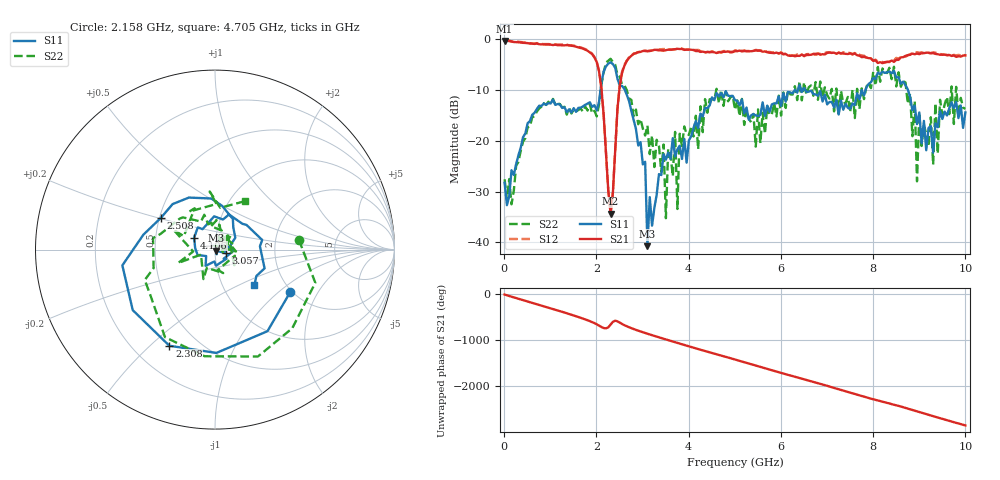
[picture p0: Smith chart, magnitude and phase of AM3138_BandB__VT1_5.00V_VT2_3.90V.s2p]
! Date/Time: Tue, Nov 13, 2018 4:40 PM
! Network Analyzer: Agilent Technologies E8364B Rev: A.07.50.67
! Sweep from 0.010 to 10.000 GHz, 201 Points, Sweep Type: LIN
! Power Supply: 5.001 V, 0.000 A
# Hz S DB R 50
!freq MagS11 AngS11 MagS21 AngS21 MagS12 AngS12 MagS22 AngS22
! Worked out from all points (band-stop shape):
!   201 points, 10 MHz to 10 GHz, reference 50 ohm
!   highest |S21| = -0.32 dB at 10 MHz (marker M1); lowest = -34.3 dB at 2.308 GHz (marker M2)
!   |S21| within 3 dB of the highest: start of sweep to 1.938 GHz; 2.751 GHz to 6.286 GHz (3.535 GHz wide, 78.2 % of centre)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
!   lowest |S11| = -40.7 dB at 3.107 GHz (marker M3), VSWR 1.02, Z = 50.7 - j0.589 ohm
!   |S11| at or under -10 dB: start of sweep to 2.089 GHz; 2.617 GHz to 6.301 GHz (3.683 GHz wide, 82.6 % of centre); 6.53 GHz to 7.836 GHz (1.307 GHz wide, 18.2 % of centre)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
!   |S22| runs from -35.2 to -3.9 dB; largest |S21 - S12| = 0.036
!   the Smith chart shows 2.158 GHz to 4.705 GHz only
!   S11 on the Smith chart (normalised r, x): 2.158 GHz: 1.97, -1.20; 2.308 GHz: 0.35, -0.58; 2.508 GHz: 0.51, +0.21; 3.057 GHz: 1.12, -0.05; 4.106 GHz: 0.79, +0.11; 4.705 GHz: 1.41, -0.61
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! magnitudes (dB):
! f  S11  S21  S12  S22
! 10 MHz  -28.2  -0.3  -0.2  -27.6
! 1.708 GHz  -13.2  -1.8  -1.8  -14.2
! 2.158 GHz  -6.4  -15.0  -14.8  -6.5
! 2.308 GHz  -4.5  -34.3  -34.2  -3.9
! 2.508 GHz  -9.1  -9.1  -8.9  -7.4
! 3.057 GHz  -24.1  -2.3  -2.2  -19.0
! 3.107 GHz  -40.7  -2.4  -2.3  -17.0
! 3.357 GHz  -26.6  -2.2  -2.0  -21.0
! 3.507 GHz  -23.7  -2.1  -1.9  -35.2
! 3.556 GHz  -22.3  -2.1  -2.1  -21.6
! 3.706 GHz  -23.1  -2.0  -2.0  -18.2
! 3.756 GHz  -21.7  -1.9  -1.9  -33.4
! 3.806 GHz  -21.0  -1.9  -1.8  -18.6
! 4.106 GHz  -17.5  -2.1  -2.1  -19.1
! 4.705 GHz  -10.6  -2.6  -2.5  -10.0
! 5.005 GHz  -12.0  -2.3  -2.2  -13.9
! 6.703 GHz  -10.8  -2.9  -2.9  -11.1
! 8.352 GHz  -6.3  -4.4  -4.5  -5.6
! 8.901 GHz  -13.0  -3.0  -2.8  -12.2
! 8.951 GHz  -16.7  -2.8  -2.6  -28.0
! 9.001 GHz  -14.4  -2.9  -2.7  -14.5
! 10 GHz  -14.4  -3.2  -3.1  -13.7
